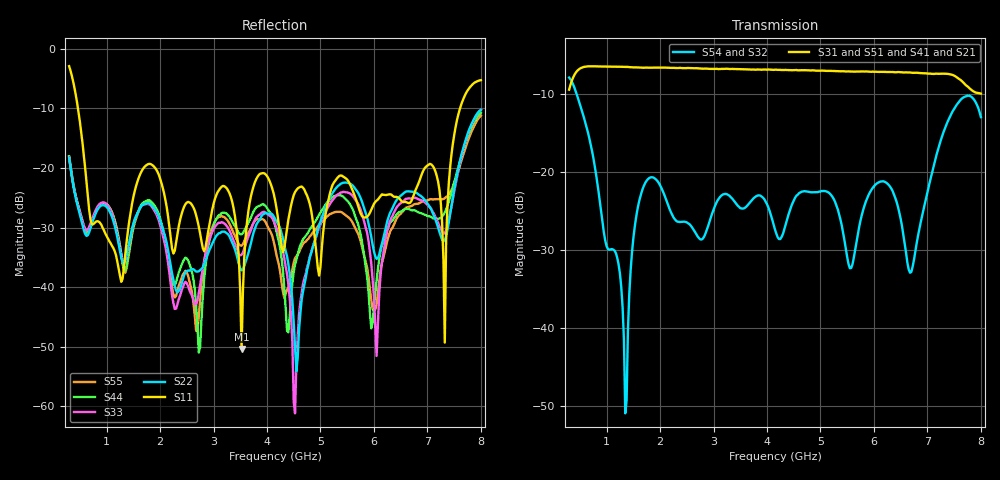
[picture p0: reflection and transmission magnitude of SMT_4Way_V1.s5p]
! Created Tue Jan 09 16:21:30 2018
# hz S ma R 50
! 5 Port Network Data from SP1.SP block
! freq  magS11  angS11  magS12  angS12  magS13  angS13  magS14  angS14
!  magS15  angS15
!  magS21  angS21  magS22  angS22  magS23  angS23
!  magS24  angS24  magS25  angS25
!  magS31  angS31  magS32  angS32
!  magS33  angS33  magS34  angS34  magS35  angS35
!  magS41  angS41
!  magS42  angS42  magS43  angS43  magS44  angS44  magS45  angS45
!  magS51  angS51  magS52  angS52  magS53  angS53  magS54  angS54
!  magS55  angS55
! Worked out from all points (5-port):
!   309 points, 300 MHz to 8 GHz, reference 50 ohm
!   strongest paths, dB at 300 MHz, 2.225 GHz, 4.15 GHz, 6.075 GHz, 8 GHz:
!     S31: -9.4, -6.6, -6.8, -7.1, -9.9
!     S51: -9.4, -6.6, -6.8, -7.2, -9.7
!     S41: -9.4, -6.6, -6.8, -7.2, -9.8
!     S21: -9.4, -6.6, -6.9, -7.2, -9.8
!     S54: -7.8, -25.4, -27.3, -21.3, -12.9
!     S32: -7.8, -25.4, -27.3, -21.3, -12.9
!   lowest |S11| = -50.4 dB at 3.525 GHz (marker M1), VSWR 1.01, Z = 50 + j0.302 ohm
!   |S11| at or under -10 dB: 464.9 MHz to 7.611 GHz (7.146 GHz wide, 177 % of centre)
